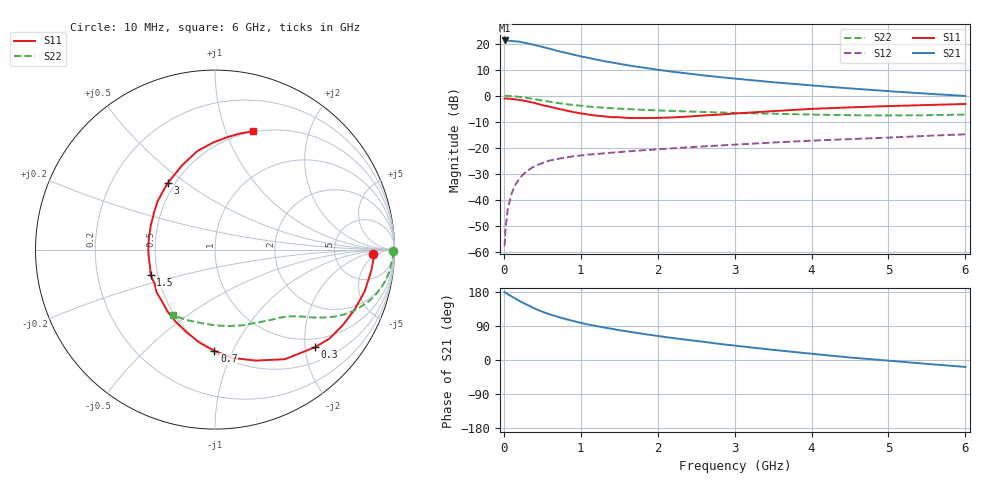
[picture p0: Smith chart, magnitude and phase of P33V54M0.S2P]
! SIEMENS Small Signal Semiconductors
! BFP181
! Si NPN RF Bipolar Junction Transistor in SOT143
! VCE = 3.5 V  IC = 4 mA
! Common Emitter S-Parameters:  March  1996
# GHz  S  MA  R  50
!  f  S11  S21  S12  S22
! GHz  MAG  ANG  MAG  ANG  MAG  ANG  MAG  ANG
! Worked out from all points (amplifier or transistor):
!   36 points, 10 MHz to 6 GHz, reference 50 ohm
!   highest |S21| = 21.2 dB at 10 MHz (marker M1)
!   |S21| within 3 dB of that: start of sweep to 572.9 MHz
!   unconditionally stable (mu >= 1): 1.887 GHz to end of sweep
!   at 250 MHz: K = 0.18, MSG = 25.3 dB, |S12| = -30.2 dB
!   at 1.4 GHz: K = 0.84, MSG = 17.3 dB, |S12| = -21.9 dB
!   at 6 GHz: K = 1.06, MAG = 5.8 dB, |S12| = -14.8 dB
!   S11 on the Smith chart (normalised r, x): 10 MHz: 15, -3; 300 MHz: 0.80, -2.21; 700 MHz: 0.52, -0.85; 1.5 GHz: 0.46, -0.15; 3 GHz: 0.46, +0.43; 6 GHz: 0.49, +1.25
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0.01  0.8793 -1.7  11.45 178.7  0.0013 78.7  0.9919 -0.6
0.02  0.8844 -3.5  11.42 177.9  0.0025 85.9  0.9947 -1.4
0.05  0.8788 -7.6  11.37 173.9  0.0067 90.8  0.9878 -3.4
0.1  0.8658 -15.6  11.21 168.0  0.0132 80.2  0.9813 -6.7
0.2  0.8273 -30.5  10.84 156.3  0.0254 73.0  0.9492 -13.0
0.25  0.8072 -38.0  10.47 150.7  0.0308 69.8  0.9275 -16.0
0.3  0.7788 -44.3  10.13 146.1  0.0359 65.9  0.9042 -18.5
0.4  0.7241 -57.5  9.4 136.0  0.0444 60.0  0.8567 -22.9
0.5  0.6589 -69.8  8.611 127.5  0.0509 54.5  0.808 -26.5
0.6  0.6118 -80.7  7.924 120.2  0.0572 50.4  0.7631 -29.3
0.7  0.5639 -90.3  7.182 114.0  0.0612 47.4  0.7237 -31.5
0.9  0.4856 -109.3  6.143 103.0  0.0687 43.1  0.6644 -34.7
1.1  0.4347 -127.4  5.305 93.4  0.074 40.2  0.6189 -37.1
1.3  0.4029 -143.8  4.603 85.8  0.0784 37.8  0.5873 -39.3
1.5  0.3861 -158.2  4.085 78.7  0.0826 36.8  0.563 -41.3
1.8  0.3721 -179.1  3.476 69.2  0.0895 35.3  0.5362 -44.5
2.2  0.3829 158.8  2.87 57.9  0.0979 33.7  0.5094 -49.4
3  0.4544 125.4  2.128 38.0  0.1151 30.4  0.467 -60.7
3.5  0.5053 111.1  1.81 26.8  0.1263 28.3  0.4506 -69.3
4.5  0.5966 91.0  1.378 6.6  0.1469 22.7  0.4226 -89.6
5.5  0.6614 77.9  1.093 -10.3  0.1697 17.9  0.4223 -111.4
6  0.6921 72.3  0.988 -18.3  0.1815 14.5  0.4342 -122.6
